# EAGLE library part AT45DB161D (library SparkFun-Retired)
16-Mbit SPI flash memory Retired IC-08556
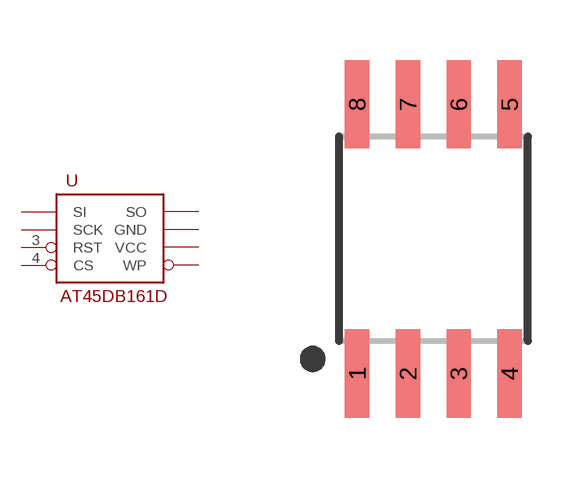
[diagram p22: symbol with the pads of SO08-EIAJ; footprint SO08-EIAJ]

Designator prefix -

## AT45DB161D  [SO08-EIAJ]
1  SI
2  SCK
3  RST
4  CS
5  WP
6  VCC
7  GND
8  SO

## Footprint SO08-EIAJ (pad centres in mm)
Fits EIAJ packages (wide version of the SOIC-8).
smd 0.61 x 2.21: 1 -1.905,-3.378; 2 -0.635,-3.378; 3 0.635,-3.378; 4 1.905,-3.378; 5 1.905,3.353; 6 0.635,3.353; 7 -0.635,3.353; 8 -1.905,3.353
